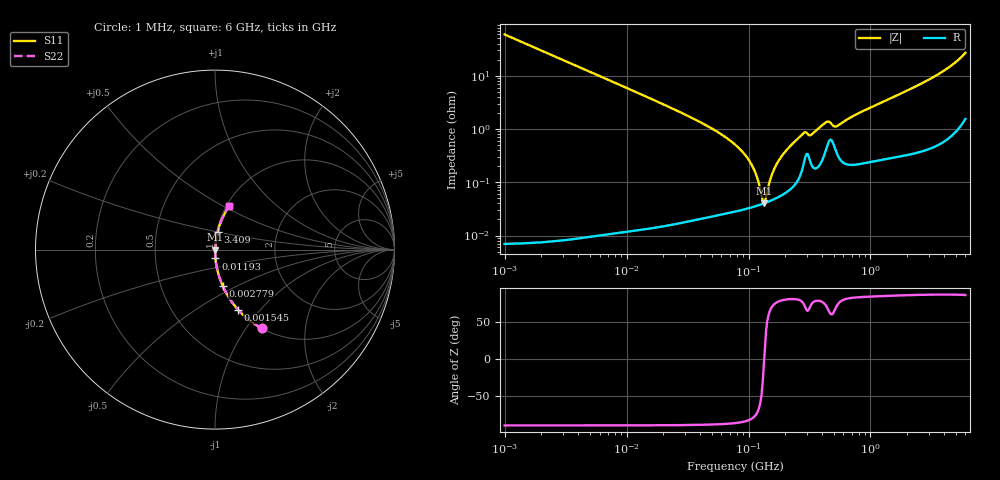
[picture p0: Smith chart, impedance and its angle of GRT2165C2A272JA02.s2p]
!Murata Part Number: GRT2165C2A272JA02
!These Parameters are Measured in Series Mode Connection
!Data Generated on Jun 19, 2026
!  o--ll--o
!Port1  Port2
!  o------o
!Operation Temp=25[degC], DC Bias Voltage=0[V]
!Freq. Start=1000[kHz] Stop=6[GHz] 401[Steps]
# Hz S RI R 50
!Freq.(Hz) S11(Real) S11(Imag) S21(Real) S21(Imag) S12(Real) S12(Imag) S22(Real) S22(Imag)
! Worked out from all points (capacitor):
!   401 points, 1 MHz to 6 GHz, reference 50 ohm
!   read as one part in series: C = 2.68 nF near 1.044 MHz
!   lowest |Z| = 40.4 mohm at 133.4 MHz (marker M1)
!   series resonance near 134.3 MHz, so ESL is about 520 pH
!   S11 on the Smith chart (normalised r, x): 1 MHz: 1.00, -1.19; 1.545 MHz: 1.00, -0.77; 2.779 MHz: 1.00, -0.43; 11.93 MHz: 1.00, -0.10; 3.409 GHz: 1.01, +0.20; 6 GHz: 1.03, +0.54
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1000000  0.2612 -0.4392  0.7388 0.4392  0.7388 0.4392  0.2612 -0.4392
1544926  0.129 -0.3351  0.871 0.3351  0.871 0.3351  0.129 -0.3351
2779283  0.0438 -0.2044  0.9562 0.2044  0.9562 0.2044  0.0438 -0.2044
4293785  0.0189 -0.1357  0.9811 0.1357  0.9811 0.1357  0.0189 -0.1357
1.193364e7  0.00256 -0.0492  0.9974 0.0492  0.9974 0.0492  0.00256 -0.0492
1.843659e7  0.00114 -0.0315  0.9989 0.0315  0.9989 0.0315  0.00114 -0.0315
4.596069e7  0.000347 -0.0114  0.9997 0.0114  0.9997 0.0114  0.000347 -0.0114
7.745967e7  0.000306 -0.0051  0.9997 0.0051  0.9997 0.0051  0.000306 -0.0051
1.073387e8  0.000344 -0.00199  0.9997 0.00199  0.9997 0.00199  0.000344 -0.00199
1.170949e8  0.000362 -0.00121  0.9996 0.00121  0.9996 0.00121  0.000362 -0.00121
1.277378e8  0.000386 -0.000442  0.9996 0.000442  0.9996 0.000442  0.000386 -0.000442
1.334167e8  0.0004 -5.67e-05  0.9996 5.67e-05  0.9996 5.67e-05  0.0004 -5.67e-05
1.39348e8  0.000415 0.000329  0.9996 -0.000329  0.9996 -0.000329  0.000415 0.000329
1.622626e8  0.000484 0.0017  0.9995 -0.0017  0.9995 -0.0017  0.000484 0.0017
1.889453e8  0.000586 0.00314  0.9994 -0.00314  0.9994 -0.00314  0.000586 0.00314
2.794814e8  0.00202 0.00793  0.998 -0.00793  0.998 -0.00793  0.00202 0.00793
3.325952e8  0.00205 0.00777  0.9979 -0.00777  0.9979 -0.00777  0.00205 0.00777
4.31778e8  0.00421 0.0126  0.9958 -0.0126  0.9958 -0.0126  0.00421 0.0126
5.251325e8  0.00375 0.0105  0.9962 -0.0105  0.9962 -0.0105  0.00375 0.0105
1.428092e9  0.00412 0.0364  0.9959 -0.0364  0.9959 -0.0364  0.00412 0.0364
3.408564e9  0.0143 0.0972  0.9857 -0.0972  0.9857 -0.0972  0.0143 0.0972
6e9  0.0797 0.2437  0.9203 -0.2437  0.9203 -0.2437  0.0797 0.2437
